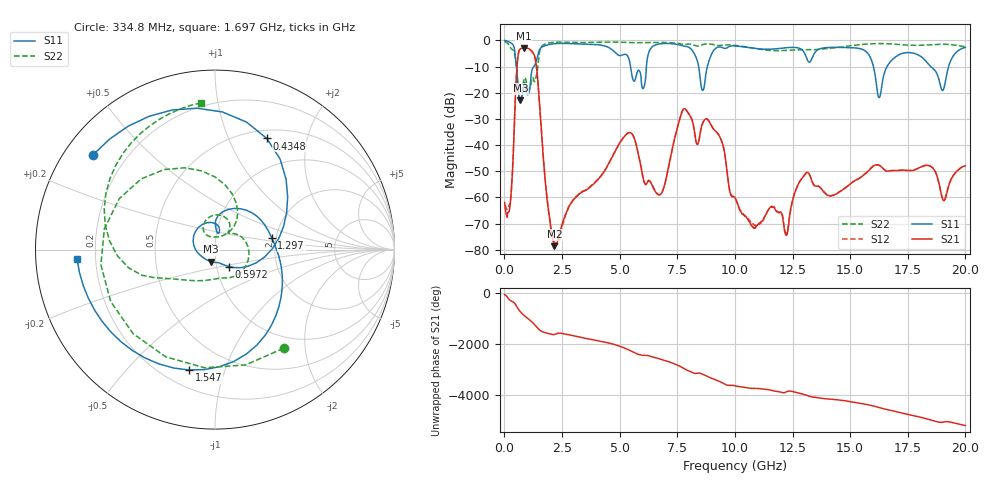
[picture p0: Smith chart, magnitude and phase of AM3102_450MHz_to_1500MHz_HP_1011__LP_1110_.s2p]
!Agilent Technologies,E8364B,MY43040894,A.07.50.67
!Agilent E8364B: A.07.50.67
!Date: Thursday, January 11, 2018 06:26:38
!Correction: S11(Full 2 Port(1,2))
!S21(Full 2 Port(1,2))
!S12(Full 2 Port(1,2))
!S22(Full 2 Port(1,2))
!S2P File: Measurements: S11, S21, S12, S22:
# Hz S  dB  R 50
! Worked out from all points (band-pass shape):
!   1601 points, 10 MHz to 20 GHz, reference 50 ohm
!   highest |S21| = -2.91 dB at 847.1 MHz (marker M1); lowest = -78.6 dB at 2.171 GHz (marker M2)
!   |S21| within 3 dB of the highest: 593.2 MHz to 1.306 GHz (712.5 MHz wide, 75 % of centre)
!   lowest |S11| = -23.0 dB at 697.2 MHz (marker M3), VSWR 1.15, Z = 47.5 - j6.49 ohm
!   |S11| at or under -10 dB: 523.2 MHz to 1.28 GHz (757.2 MHz wide, 84 % of centre); 5.474 GHz to 6.162 GHz (687.7 MHz wide, 11.8 % of centre); 18.5 GHz to 19.27 GHz (777.2 MHz wide, 4.12 % of centre)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
!   |S22| runs from -23.1 to -0.5 dB; largest |S21 - S12| = 0.0009
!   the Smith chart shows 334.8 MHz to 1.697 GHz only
!   S11 on the Smith chart (normalised r, x): 334.8 MHz: 0.08, +0.34; 434.8 MHz: 0.60, +1.39; 597.2 MHz: 1.14, -0.22; 1.297 GHz: 1.90, +0.27; 1.547 GHz: 0.30, -0.76; 1.697 GHz: 0.13, -0.03
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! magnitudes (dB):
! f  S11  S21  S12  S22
! 10 MHz  -0.1  -61.9  -62.9  -0.5
! 334.8 MHz  -1.3  -52.9  -52.7  -3.5
! 434.8 MHz  -3.3  -31.5  -31.5  -4.4
! 597.2 MHz  -18.3  -5.6  -5.6  -18.6
! 697.2 MHz  -23.0  -3.2  -3.2  -23.1
! 847.1 MHz  -16.5  -2.9  -2.9  -15.0
! 1.297 GHz  -9.8  -5.7  -5.7  -15.8
! 1.547 GHz  -3.3  -27.4  -27.4  -3.6
! 1.697 GHz  -2.3  -45.7  -45.6  -1.7
! 2.171 GHz  -1.3  -78.6  -77.7  -0.8
! 3.346 GHz  -1.4  -58.1  -57.9  -0.8
! 5.432 GHz  -8.1  -35.2  -35.2  -0.9
! 6.032 GHz  -18.3  -53.2  -53.1  -0.9
! 6.682 GHz  -1.4  -59.0  -58.8  -0.8
! 7.819 GHz  -2.3  -26.1  -26.1  -1.6
! 8.606 GHz  -19.1  -31.6  -31.6  -1.6
! 10.01 GHz  -2.1  -60.1  -60.2  -1.9
! 12.23 GHz  -2.8  -74.5  -73.8  -3.8
! 13.34 GHz  -7.0  -53.7  -53.7  -3.6
! 16.68 GHz  -9.0  -49.9  -50.0  -1.3
! 19.01 GHz  -19.2  -60.6  -60.5  -1.5
! 20 GHz  -2.7  -47.9  -47.9  -2.4
